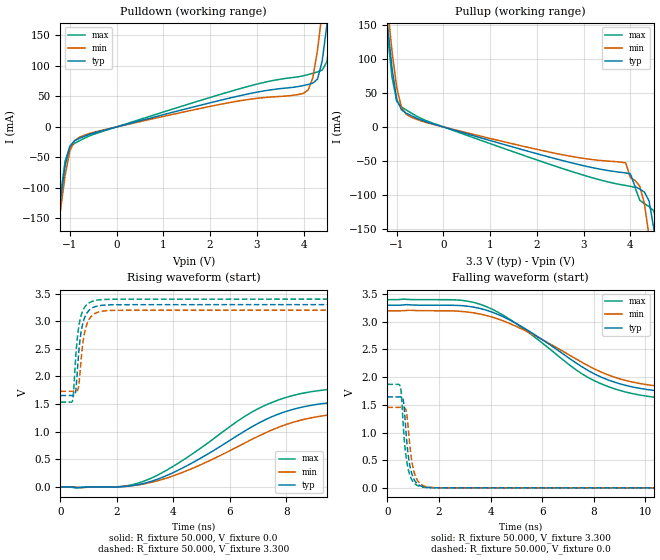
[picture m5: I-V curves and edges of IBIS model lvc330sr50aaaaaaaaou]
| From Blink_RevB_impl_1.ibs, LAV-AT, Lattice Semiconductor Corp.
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[Model] lvc330sr50aaaaaaaaou
Model_type Output
Polarity   Non-Inverting
Enable   Active-High
Vmeas =  1.650V
Cref =  0.0F
Rref =  1.000M
Vref =  0.0V
C_comp   2.000pF   1.500pF   2.500pF
[Temperature Range]   25.000   0.125k   -40.000
[Voltage Range]   3.300V   3.200V   3.400V
[C Comp Corner]
C_comp   2.000pF   1.500pF   2.500pF
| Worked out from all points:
|   slope of the pulldown table from 0 to 0.495 V, typ, clamps not added: 49.7 ohm
|   slope of the pullup table from 0 to 0.495 V, typ, clamps not added: 49.7 ohm
|   rising waveform, R_fixture 50.000, V_fixture 0.0: 20-80 % time 3.44ns typ, 3.74ns min, 3.34ns max; typ from 0 V to 1.65 V
|   rising waveform, R_fixture 50.000, V_fixture 3.300: 20-80 % time 216ps typ, 226ps min, 208ps max; typ from 1.66 V to 3.3 V
|   falling waveform, R_fixture 50.000, V_fixture 3.300: 20-80 % time 3.39ns typ, 3.6ns min, 3.34ns max; typ from 3.3 V to 1.65 V
|   falling waveform, R_fixture 50.000, V_fixture 0.0: 20-80 % time 230ps typ, 241ps min, 222ps max; typ from 1.64 V to 0 V
[Pulldown]
|Voltage   I(typ)   I(min)   I(max)
-3.3V     -1.863A    -1.857A    -1.871A
-1.3V     -190.1mA   -204.9mA   -183.4mA
-1.1V     -63.12mA   -79.3mA    -55.91mA
-900mV    -22.81mA   -22.66mA   -27.09mA
-700mV    -15.71mA   -13.84mA   -19.04mA
4V        67.86mA    55.12mA    83.89mA
4.2V      71.79mA    80.69mA    87.95mA
4.4V      108mA      189.4mA    93.09mA
4.5V      167mA      262.8mA    106.8mA
4.6V      240.7mA    341.7mA    156.9mA
4.7V      321mA      424mA      229.7mA
6.6V      2.037A     2.132A     1.946A
[Pullup]
|Voltage   I(typ)   I(min)   I(max)
-3.3V     2.034A     2.037A     2.035A
-1.2V     153.9mA    179.6mA    139.6mA
-1.1V     86.54mA    111.8mA    73.31mA
-1V       41.19mA    58.71mA    37.84mA
-800mV    20.49mA    18.8mA     25.14mA
3.9V      -67.85mA   -52.92mA   -86.29mA
4.1V      -87.88mA   -78.73mA   -89.23mA
4.2V      -91.53mA   -87.37mA   -107.9mA
4.4V      -109mA     -160.9mA   -117.4mA
4.5V      -149.1mA   -223.5mA   -123.6mA
4.6V      -211mA     -293.7mA   -150.3mA
6.6V      -1.873A    -1.951A    -1.796A
[Ramp]
| variable   typ   min   max
dV/dt_r   0.133u/0.102p   0.169u/0.364p   0.571u/0.408p
dV/dt_f   0.540u/0.300p   1.740u/1.024p   60.000n/4.819f
R_load = 50.000
[Rising Waveform]
R_fixture= 50.000
V_fixture= 0.0
V_fixture_min= 0.0
V_fixture_max= 0.0
|time   V(typ)   V(min)   V(max)
0s        2.499uV    9.523uV    928.8nV
2.09ns    2.904mV    4.902mV    6.716mV
2.94ns    63.58mV    55.05mV    102.8mV
4.36ns    352.3mV    271.3mV    491.9mV
6.3ns     940.4mV    735mV      1.2V
7.17ns    1.195V     957.7mV    1.458V
8.36ns    1.421V     1.189V     1.672V
9.95ns    1.545V     1.33V      1.783V
16.49ns   1.636V     1.444V     1.861V
50ns      1.645V     1.456V     1.871V
[Rising Waveform]
R_fixture= 50.000
V_fixture= 3.300
V_fixture_min= 3.200
V_fixture_max= 3.400
|time   V(typ)   V(min)   V(max)
0s        1.655V     1.732V     1.536V
430ps     1.656V     1.733V     1.565V
460ps     1.654V     1.733V     1.686V
540ps     1.734V     1.732V     2.343V
630ps     2.322V     1.784V     2.833V
780ps     2.932V     2.545V     3.174V
880ps     3.093V     2.847V     3.268V
1ns       3.19V      3.019V     3.328V
1.45ns    3.287V     3.179V     3.391V
50ns      3.3V       3.2V       3.4V
[Falling Waveform]
R_fixture= 50.000
V_fixture= 3.300
V_fixture_min= 3.200
V_fixture_max= 3.400
|time   V(typ)   V(min)   V(max)
0s        3.3V       3.2V       3.4V
2.71ns    3.296V     3.193V     3.394V
3.63ns    3.237V     3.137V     3.311V
5.06ns    2.952V     2.903V     2.946V
7.23ns    2.282V     2.351V     2.16V
7.97ns    2.071V     2.162V     1.948V
9.2ns     1.856V     1.944V     1.736V
10.87ns   1.735V     1.82V      1.615V
16.86ns   1.662V     1.739V     1.544V
50ns      1.654V     1.73V      1.535V
[Falling Waveform]
R_fixture= 50.000
V_fixture= 0.0
V_fixture_min= 0.0
V_fixture_max= 0.0
|time   V(typ)   V(min)   V(max)
0s        1.644V     1.454V     1.87V
500ps     1.644V     1.454V     1.835V
550ps     1.642V     1.455V     1.647V
620ps     1.576V     1.455V     1.108V
700ps     1.161V     1.429V     665.2mV
810ps     588.9mV    1.079V     337mV
960ps     239.3mV    451.9mV    137.6mV
1.15ns    79.78mV    149.1mV    46.18mV
1.49ns    12.21mV    22.43mV    7.305mV
50ns      1.835uV    9.11uV     -383nV
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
